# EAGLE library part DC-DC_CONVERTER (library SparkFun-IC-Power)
APTS006A0X-SRZ (IC-09258) Step-down 6A variable voltage switching module (TOL-09275)
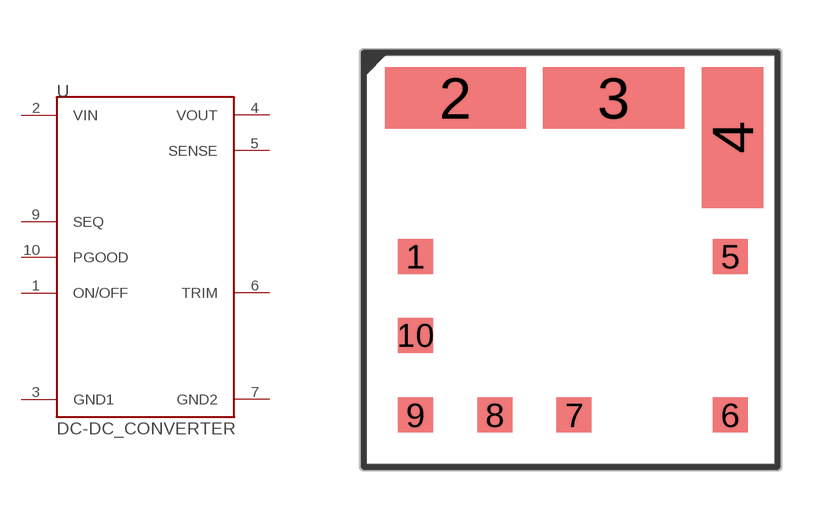
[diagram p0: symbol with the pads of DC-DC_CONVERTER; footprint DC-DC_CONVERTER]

Designator prefix -

## DC-DC_CONVERTER  [DC-DC_CONVERTER]
1  ON/OFF
2  VIN
3  GND1
4  VOUT
5  SENSE
6  TRIM
7  GND2
9  SEQ
10  PGOOD

## Footprint DC-DC_CONVERTER (pad centres in mm)
smd 1.01 x 1.01: 1 -4.48,0.1; 5 4.61,0.1; 6 4.61,-4.48; 7 0.1,-4.48; 8 -2.19,-4.48; 9 -4.48,-4.48; 10 -4.48,-2.19
smd 4.07 x 1.77: 2 -3.33,4.67; 3 1.24,4.67
smd 1.77 x 4.07: 4 4.67,3.53

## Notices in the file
Licensing: Creative Commons ShareAlike 4.0 International - https://creativecommons.org/licenses/by-sa/4.0
